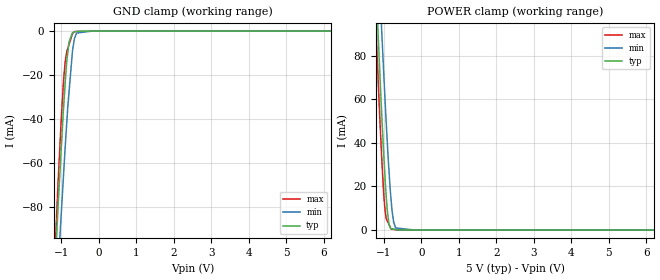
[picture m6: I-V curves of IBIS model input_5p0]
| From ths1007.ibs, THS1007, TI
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|   input_5p0 Model
[Model]   input_5p0
Model_type   Input
Vinl = 0.6
Vinh = 2.6
|   typ   min   max
|   (nom PVT)   (fast PVT)   (slow PVT)
C_comp   9.560e-13   9.523e-13   9.597e-13
| Where nom  PVT is Nominal Process, 5V, 27C
| Fast PVT is Strong Process,  5.25V, -40C
| Slow PVT is Weak Process,   4.75V, 125C
[Voltage Range]   5   4.75   5.25
|Ambient Temperature   25   85   -40
|Junction Temperature
[Temperature Range]   27   125   -40
[Power Clamp Reference]   5   4.75   5.25
[GND Clamp Reference]   0   0   0
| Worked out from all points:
|   GND clamp passes 1 mA (typ) near -0.71 V on its own axis
|   POWER clamp passes 1 mA (typ) near -0.83 V on its own axis
[GND Clamp]
|   Voltage   I(typ)   I(min)   I(max)
-5V       -1.675A    -1.596A    -1.773A
-1.306V   -155.6mA   -179.1mA   -152.8mA
-1.088V   -80.06mA   -108.9mA   -69.56mA
-1.031V   -62.21mA   -91.46mA   -49.88mA
-934.5mV  -33.25mA   -63.59mA   -21.15mA
-855mV    -13.72mA   -41.54mA   -9.273mA
-795mV    -4.976mA   -27.9mA    -6.115mA
-703mV    -917.7uA   -9.165mA   -1.272mA
-640mV    -213.3uA   -2.99mA    -237.7uA
-593.8mV  -169.5uA   -911.3uA   -220.5uA
-190mV    0A         -23.35nA   -70.56uA
10V       0A         0A         0A
[POWER Clamp]
|   Voltage   I(typ)   I(min)   I(max)
-5V       1.776A     1.782A     1.785A
-1.306V   150.2mA    188mA      131.4mA
-1.113V   74.6mA     113mA      53.59mA
-1.054V   52.58mA    90.92mA    32.57mA
-966mV    23.56mA    59.37mA    8.827mA
-910mV    9.312mA    41.17mA    4.274mA
-860mV    2.445mA    26.65mA    2.447mA
-803.3mV  599.5uA    13.29mA    372.2uA
-736.2mV  359.7uA    3.523mA    231.3uA
-684mV    172.7uA    932.3uA    121.4uA
-190mV    0A         0A         8.884uA
10V       0A         0A         0A
